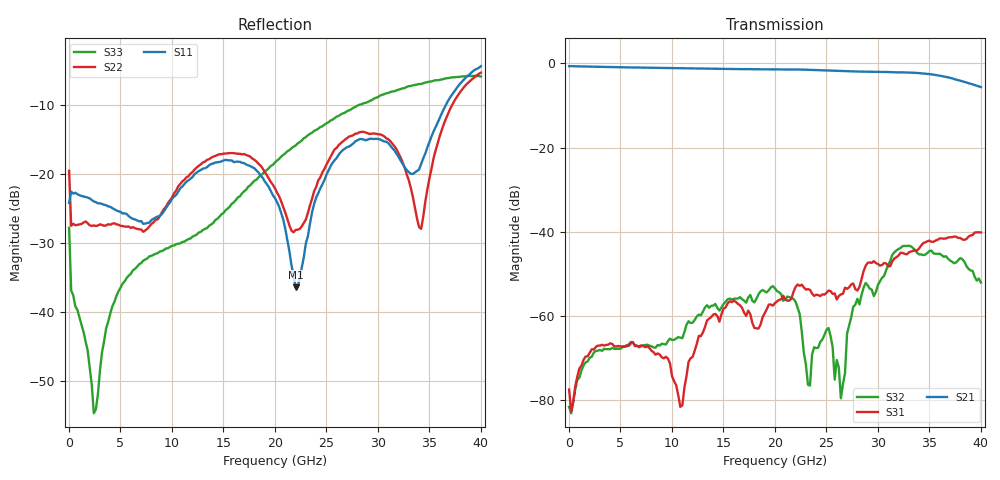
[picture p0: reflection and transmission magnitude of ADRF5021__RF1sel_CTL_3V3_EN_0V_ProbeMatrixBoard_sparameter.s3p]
! Device:  ADRF5021
! Description: SOI MMIC SPDT Non-Reflective Switch
! Frequency:  9 kHz -  30 GHz
! Ports:
! 	RFC	= Port 1
!	RF1	= Port 2
!	RF2	= Port 3
! Vdd:  +3.3 Volt
! Vss:  -2.5 Volt
! Control:  0/+3.3 Volt
! State:  RF1 Selected (Vctl= +3.3 V, Ven= 0 V)
! Data:  The device was measured using G-S-G Probes on a matrix board.
!  Data was collected using an calibrated 4 port network analyzer.
!  The reference plane is the package pins of ADRF5021 switch.
! Note:  Analog Devices supplies this data as a sample of measured data at the package pin
!  for this product.  Your particular data for this product may vary.
!  Data was taken at 25 degrees C.
!  Analog Devices reserves the right to change this data at anytime.
# GHZ S DB R 50.0
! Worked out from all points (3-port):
!   201 points, 10 MHz to 40.01 GHz, reference 50 ohm
!   strongest paths, dB at 10 MHz, 10.01 GHz, 20.01 GHz, 30.01 GHz, 40.01 GHz:
!     S21: -0.7, -1.1, -1.4, -2.0, -5.6
!     S31: -77.4, -74.3, -56.9, -47.6, -40.1
!     S32: -81.6, -65.7, -53.5, -52.6, -52.0
!   lowest |S11| = -36.4 dB at 22.01 GHz (marker M1), VSWR 1.03, Z = 49.5 - j1.42 ohm
!   |S11| at or under -10 dB: start of sweep to 36.6 GHz
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0.01  -24.18 73.4  -0.67 0.6  -86.83 56.1
      -0.67 0.3  -19.53 69.7  -80.07 -169.4
      -77.44 102.2  -81.58 93.4  -27.79 -65.4
2.41  -23.97 -43.9  -0.77 -29.1  -67.68 42.0
      -0.77 -29.0  -27.44 -54.3  -68.64 30.7
      -67.94 43.6  -68.66 28.6  -54.70 93.3
11.01  -21.78 -60.1  -1.15 -129.7  -80.31 -24.8
       -1.15 -129.7  -21.05 -63.4  -65.30 -101.1
       -81.23 -17.2  -65.24 -98.2  -29.86 -69.1
20.01  -23.51 -141.2  -1.42 124.0  -57.14 117.9
       -1.41 124.2  -22.07 -135.5  -53.34 58.0
       -56.91 117.4  -53.45 56.7  -18.31 -40.5
22.01  -36.45 -108.2  -1.44 99.6  -52.93 117.2
       -1.45 99.6  -28.11 -93.6  -56.88 6.4
       -53.09 117.9  -56.61 9.2  -15.86 -43.4
26.41  -16.80 -50.9  -1.79 45.2  -54.82 112.1
       -1.81 45.3  -15.51 -59.3  -78.70 111.2
       -54.85 112.4  -79.53 92.3  -11.34 -54.8
27.61  -15.56 -62.6  -1.90 30.2  -52.19 111.5
       -1.92 30.3  -14.36 -71.8  -57.94 173.6
       -52.27 112.8  -57.80 172.0  -10.39 -58.9
31.81  -17.04 -93.7  -2.11 -23.5  -46.01 103.3
       -2.12 -23.4  -16.39 -110.1  -44.43 115.4
       -46.01 103.2  -44.42 115.5  -7.85 -74.1
34.21  -18.54 -44.1  -2.36 -57.5  -43.33 90.1
       -2.34 -57.3  -27.94 -50.1  -45.37 63.0
       -43.25 90.4  -45.36 62.6  -6.94 -83.9
40.01  -4.34 -68.3  -5.63 -139.7  -40.16 35.1
       -5.62 -139.5  -5.29 -56.6  -52.29 35.9
       -40.14 35.0  -52.03 37.6  -5.85 -109.0
